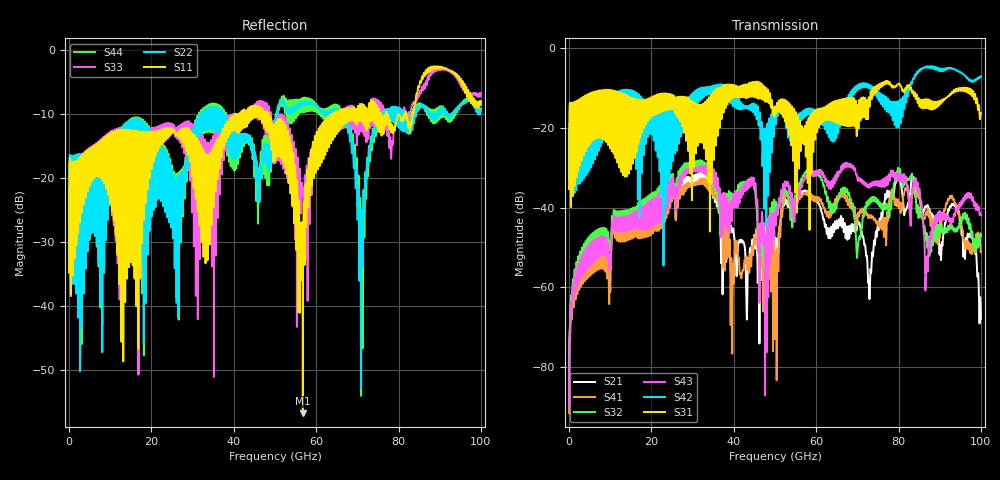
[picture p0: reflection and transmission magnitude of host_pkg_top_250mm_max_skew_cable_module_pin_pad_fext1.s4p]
# Hz S RI R 50
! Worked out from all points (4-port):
!   10000 points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, 10 MHz to 100 GHz, reference 50 ohm
!   strongest paths, dB at 10 MHz, 25.01 GHz, 50.01 GHz, 75.01 GHz, 100 GHz:
!     S31: -35.3, -11.6, -14.8, -9.2, -16.3
!     S42: -35.3, -14.4, -15.0, -11.9, -7.0
!     S43: -90.4, -37.2, -41.1, -33.6, -41.9
!     S32: -88.7, -35.8, -40.3, -38.3, -47.2
!     S41: -91.7, -38.4, -73.1, -44.5, -51.2
!     S21: -89.8, -37.2, -53.5, -44.3, -68.0
!   lowest |S11| = -56.8 dB at 56.76 GHz (marker M1), VSWR 1.00, Z = 50.1 - j0.0894 ohm
!   |S11| at or under -10 dB: start of sweep to 40.64 GHz; 48.51 GHz to 63.8 GHz (15.29 GHz wide, 27.2 % of centre); 77.1 GHz to 79.88 GHz (2.778 GHz wide, 3.54 % of centre)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
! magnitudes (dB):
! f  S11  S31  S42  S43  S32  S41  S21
! 10 MHz  -34.8  -35.3  -35.3  -90.4  -88.7  -91.7  -89.8
! 10.91 GHz  -19.9  -16.3  -11.8  -42.3  -40.8  -44.2  -42.8
! 49.98 GHz  -14.6  -15.2  -15.4  -41.1  -40.0  -65.8  -52.2
! 56.76 GHz  -56.8  -21.7  -16.2  -33.3  -32.0  -36.7  -35.8
! 70.88 GHz  -11.1  -13.4  -9.9  -33.0  -45.2  -41.3  -45.5
! 93.37 GHz  -3.5  -10.6  -5.1  -42.2  -45.5  -37.8  -39.0
! 100 GHz  -8.0  -16.3  -7.0  -41.9  -47.2  -51.2  -68.0
